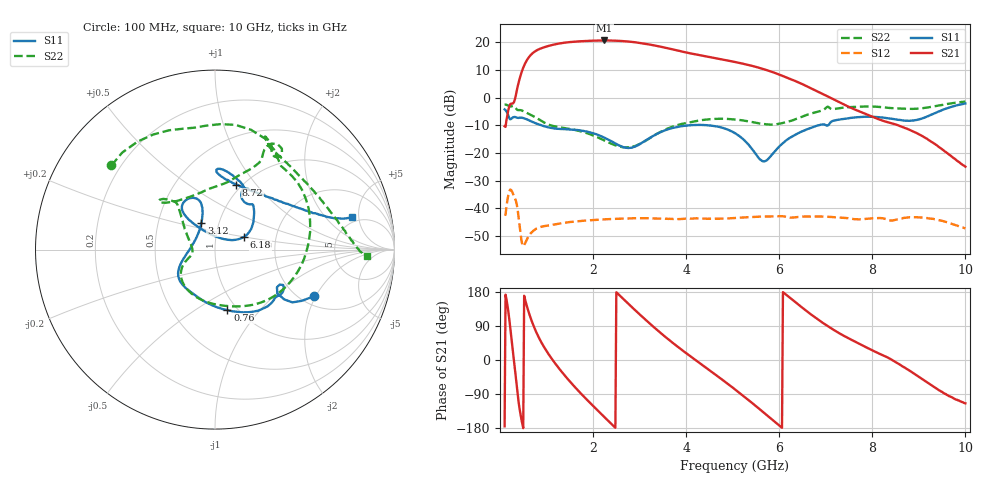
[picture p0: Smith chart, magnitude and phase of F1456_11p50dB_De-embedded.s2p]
! Integrated Device Technology
! Corporate Headquarters
! 6024 Silver Creek Valley Road
! San Jose, CA 95138  USA
! Phone:  1-408-284-8200
! Toll Free:  1-800-223-1366
! Webpage:  http://www.idt.com/
! Timing and RF Division
! 515 Groton Road, Suite 102
! Westford, MA 01886-6024
! Device:  F1456
! Description: 6-bit 0.5 dB Transmit Variable Gain Amplifier
! Frequency:  2100.0 -  2950.00 MHz
! Package:  6x6 mm Thin QFN Plastic Package: 28 pin
! State:  23
! Atten State:  11.5 dB
! Voltage:  +5.00 Volts
! Current:  217.001 mA
! Data:  The device was measured on a the F1455 evaluation board which has
!  individual transmission lines to the RF pins.  Data was collected
!  using a calibrated network analyzer.  The evaluation board was
!  de-embedded using a TRL calibration technique.
!  The reference plane is the edge of the package pin.
!  Pin  1 = CSb
!  Pin  2 = DATA
!  Pin  3 = CLK
!  Pin  4 = RSET
!  Pin  5 = GND
!  Pin  6 = RFIN  = Port 1
!  Pin  7 = GND
!  Pin  8 = NC
!  Pin  9 = NC
!  Pin 10 = NC
!  Pin 11 = NC
!  Pin 12 = NC
!  Pin 13 = NC
!  Pin 14 = /STBY
!  Pin 15 = GND
!  Pin 16 = RFOUT  = Port 2
!  Pin 17 = GND
!  Pin 18 = NC
!  Pin 19 = NC
!  Pin 20 = NC
!  Pin 21 = GND
!  Pin 22 = NC
!  Pin 23 = GND
!  Pin 24 = NC
!  Pin 25 = NC
!  Pin 26 = NC
!  Pin 27 = GND
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# GHz S dB R 50
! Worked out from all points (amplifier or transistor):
!   496 points, 100 MHz to 10 GHz, reference 50 ohm
!   highest |S21| = 20.6 dB at 2.24 GHz (marker M1)
!   |S21| within 3 dB of that: 860.7 MHz to 3.651 GHz (2.79 GHz wide, 124 % of centre)
!   unconditionally stable (mu >= 1): start of sweep to end of sweep
!   at 1.74 GHz: K = 7.28, MAG = 20.9 dB, |S12| = -44.6 dB
!   at 5.06 GHz: K = 13.74, MAG = 13.8 dB, |S12| = -43.5 dB
!   at 10 GHz: K = 230.23, MAG = -15.5 dB, |S12| = -47.3 dB
!   S11 on the Smith chart (normalised r, x): 100 MHz: 2.35, -1.95; 760 MHz: 0.90, -0.69; 3.12 GHz: 0.82, +0.25; 6.18 GHz: 1.37, +0.20; 8.72 GHz: 0.94, +0.80; 10 GHz: 4.32, +4.02
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0.1  -4.28 -25.2  -10.37 -175.2  -42.31 46.6  -2.57 140.9
0.32  -7.02 -32.7  -0.73 -21.6  -36.39 -141.9  -3.37 65.7
0.44  -7.28 -42.8  7.82 -142.5  -48.92 140.2  -4.54 38.9
0.58  -7.89 -59.3  13.56 141.4  -51.21 171.4  -5.55 6.3
0.76  -9.28 -78.3  16.77 79.0  -47.64 132.3  -7.13 -30.0
0.98  -10.50 -99.7  18.35 27.8  -46.41 91.8  -9.30 -67.4
1.2  -11.24 -116.7  19.31 -11.3  -45.82 66.5  -10.49 -95.5
1.5  -11.52 -133.8  20.05 -56.5  -45.02 40.7  -11.35 -124.6
1.76  -11.96 -144.4  20.39 -91.1  -44.60 22.9  -12.31 -141.3
2.24  -14.47 -162.2  20.65 -150.2  -44.05 -4.9  -15.49 -159.7
2.62  -17.76 169.8  20.45 164.6  -43.79 -24.9  -17.93 -171.7
3.12  -15.66 117.5  19.45 107.1  -43.63 -50.5  -15.74 156.3
3.4  -12.91 107.9  18.57 76.8  -43.74 -63.8  -12.90 140.9
4.08  -10.01 114.0  16.02 11.0  -43.79 -93.1  -8.98 130.8
4.6  -10.27 126.8  14.32 -35.9  -43.85 -115.7  -7.72 137.0
5.06  -12.98 131.2  12.82 -78.5  -43.54 -135.4  -7.92 138.9
5.64  -23.01 80.1  10.40 -136.0  -43.07 -166.7  -9.54 122.8
6.18  -15.10 23.6  7.07 169.2  -43.26 160.3  -8.74 84.0
6.7  -10.84 40.8  3.24 118.7  -43.00 133.1  -5.72 64.3
8.36  -7.52 87.2  -9.02 4.7  -44.40 62.7  -3.75 62.4
8.72  -8.38 71.8  -11.10 -22.1  -43.45 54.4  -4.05 50.3
10  -2.14 13.4  -25.00 -114.4  -47.35 -26.9  -1.46 -2.6
